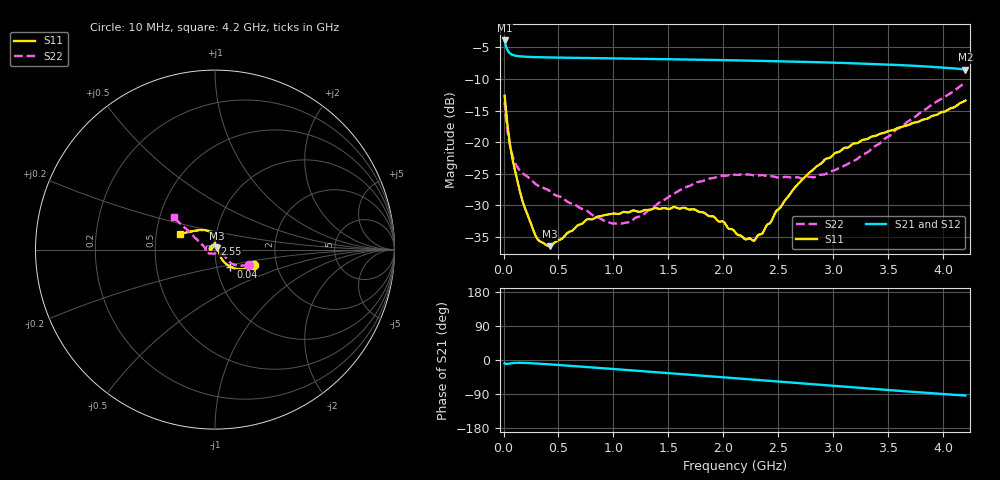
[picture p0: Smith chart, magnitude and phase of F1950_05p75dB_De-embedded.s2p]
! Integrated Device Technology
! Corporate Headquarters
! 6024 Silver Creek Valley Road
! San Jose, CA 95138  USA
! Phone:  1-408-284-8200
! Toll Free:  1-800-223-1366
! Webpage:  http://www.idt.com/
! Timing and RF Division
! 515 Groton Road, Suite 102
! Westford, MA 01886-6024
! Device:  F1950
! Description: 7-bit 0.25 dB Digital Step Attenuator
! Frequency:  150.0 -  4000.00 MHz
! Package:  4x4 mm Thin QFN Plastic Package: 24 pin
! Ports:  2 RF, 12 DC
!  Pin  1  = D0
!  Pin  2  = VDD
!  Pin  3  = Vmode
!  Pin  4  = GND
!  Pin  5  = RF1  =  Port 1
!  Pin  6  = GND
!  Pin  7  = GND
!  Pin  8  = GND
!  Pin  9  = GND
!  Pin 10  = GND
!  Pin 11  = GND
!  Pin 12  = GND
!  Pin 13  = GND
!  Pin 14  = RF2  =  Port 2
!  Pin 15  = GND
!  Pin 16  = LE
!  Pin 17  = CLK
!  Pin 18  = DATE
!  Pin 19  = D6
!  Pin 20  = D5
!  Pin 21  = D4
!  Pin 22  = D3
!  Pin 23  = D2
!  Pin 24  = D1
! State:  23
! Atten State:  5.75 dB
! Voltage:  +5.00 Volts
! Current:  Not Measured mA
! Data:  The device was measured on a the F195X evaluation board which has
!  individual transmission lines to the RF pins.  Data was collected
!  using a calibrated network analyzer.  The evaluation board was
!  de-embedded using a TRL calibration technique.
!  The reference plane is the edge of the package pin.
! Misc:  Board 2019
!  Action Tracker AT0250
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# GHz S dB R 50
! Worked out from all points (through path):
!   420 points, 10 MHz to 4.2 GHz, reference 50 ohm
!   highest |S21| = -3.93 dB at 10 MHz (marker M1); lowest = -8.5 dB at 4.2 GHz (marker M2)
!   group delay of S21, straight-line fit = 60.4 ps
!   lowest |S11| = -36.4 dB at 420 MHz (marker M3), VSWR 1.03, Z = 51.3 + j0.862 ohm
!   |S11| at or under -10 dB: start of sweep to end of sweep
!   |S22| runs from -32.9 to -10.6 dB; largest |S21 - S12| = 0.00053
!   S11 on the Smith chart (normalised r, x): 10 MHz: 1.52, -0.28; 40 MHz: 1.16, -0.22; 2.55 GHz: 0.99, +0.07; 4.2 GHz: 0.67, +0.13
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0.01  -12.66 -22.1  -3.93 -8.4  -3.92 -8.4  -13.59 -24.2
0.04  -17.87 -48.0  -5.58 -10.0  -5.58 -10.0  -18.69 -40.1
0.07  -21.57 -53.9  -6.10 -8.4  -6.10 -8.4  -21.39 -38.7
0.1  -24.15 -54.1  -6.30 -7.6  -6.30 -7.6  -23.03 -34.7
0.19  -30.18 -38.2  -6.49 -7.7  -6.49 -7.7  -25.13 -32.7
0.31  -35.32 -5.3  -6.57 -9.4  -6.57 -9.4  -26.82 -32.0
0.42  -36.43 33.9  -6.61 -11.5  -6.61 -11.5  -27.70 -32.4
0.71  -32.92 94.1  -6.69 -17.5  -6.69 -17.5  -30.51 -45.2
0.93  -31.47 116.5  -6.74 -22.2  -6.74 -22.3  -32.53 -67.9
1.05  -31.34 126.9  -6.77 -24.8  -6.77 -24.8  -32.91 -88.7
1.26  -30.89 145.2  -6.82 -29.4  -6.82 -29.4  -31.61 -121.3
1.41  -30.51 158.8  -6.86 -32.7  -6.86 -32.7  -29.61 -138.2
1.74  -30.65 178.3  -6.95 -40.0  -6.95 -40.0  -26.46 -158.5
2  -32.56 176.8  -7.03 -45.7  -7.03 -45.8  -25.31 -167.5
2.11  -34.29 169.7  -7.07 -48.2  -7.07 -48.2  -25.16 -170.3
2.28  -35.55 133.4  -7.13 -51.9  -7.13 -52.0  -25.26 -173.6
2.36  -34.26 117.0  -7.16 -53.7  -7.16 -53.8  -25.22 -175.3
2.55  -29.42 93.9  -7.23 -57.9  -7.23 -58.0  -25.51 -179.8
2.81  -24.42 90.7  -7.34 -63.8  -7.34 -63.8  -25.55 173.1
3.19  -20.19 102.8  -7.54 -72.4  -7.53 -72.4  -22.92 161.0
3.51  -18.20 118.2  -7.74 -79.5  -7.74 -79.5  -19.01 151.2
4.2  -13.41 155.2  -8.52 -93.6  -8.51 -93.7  -10.64 141.8
